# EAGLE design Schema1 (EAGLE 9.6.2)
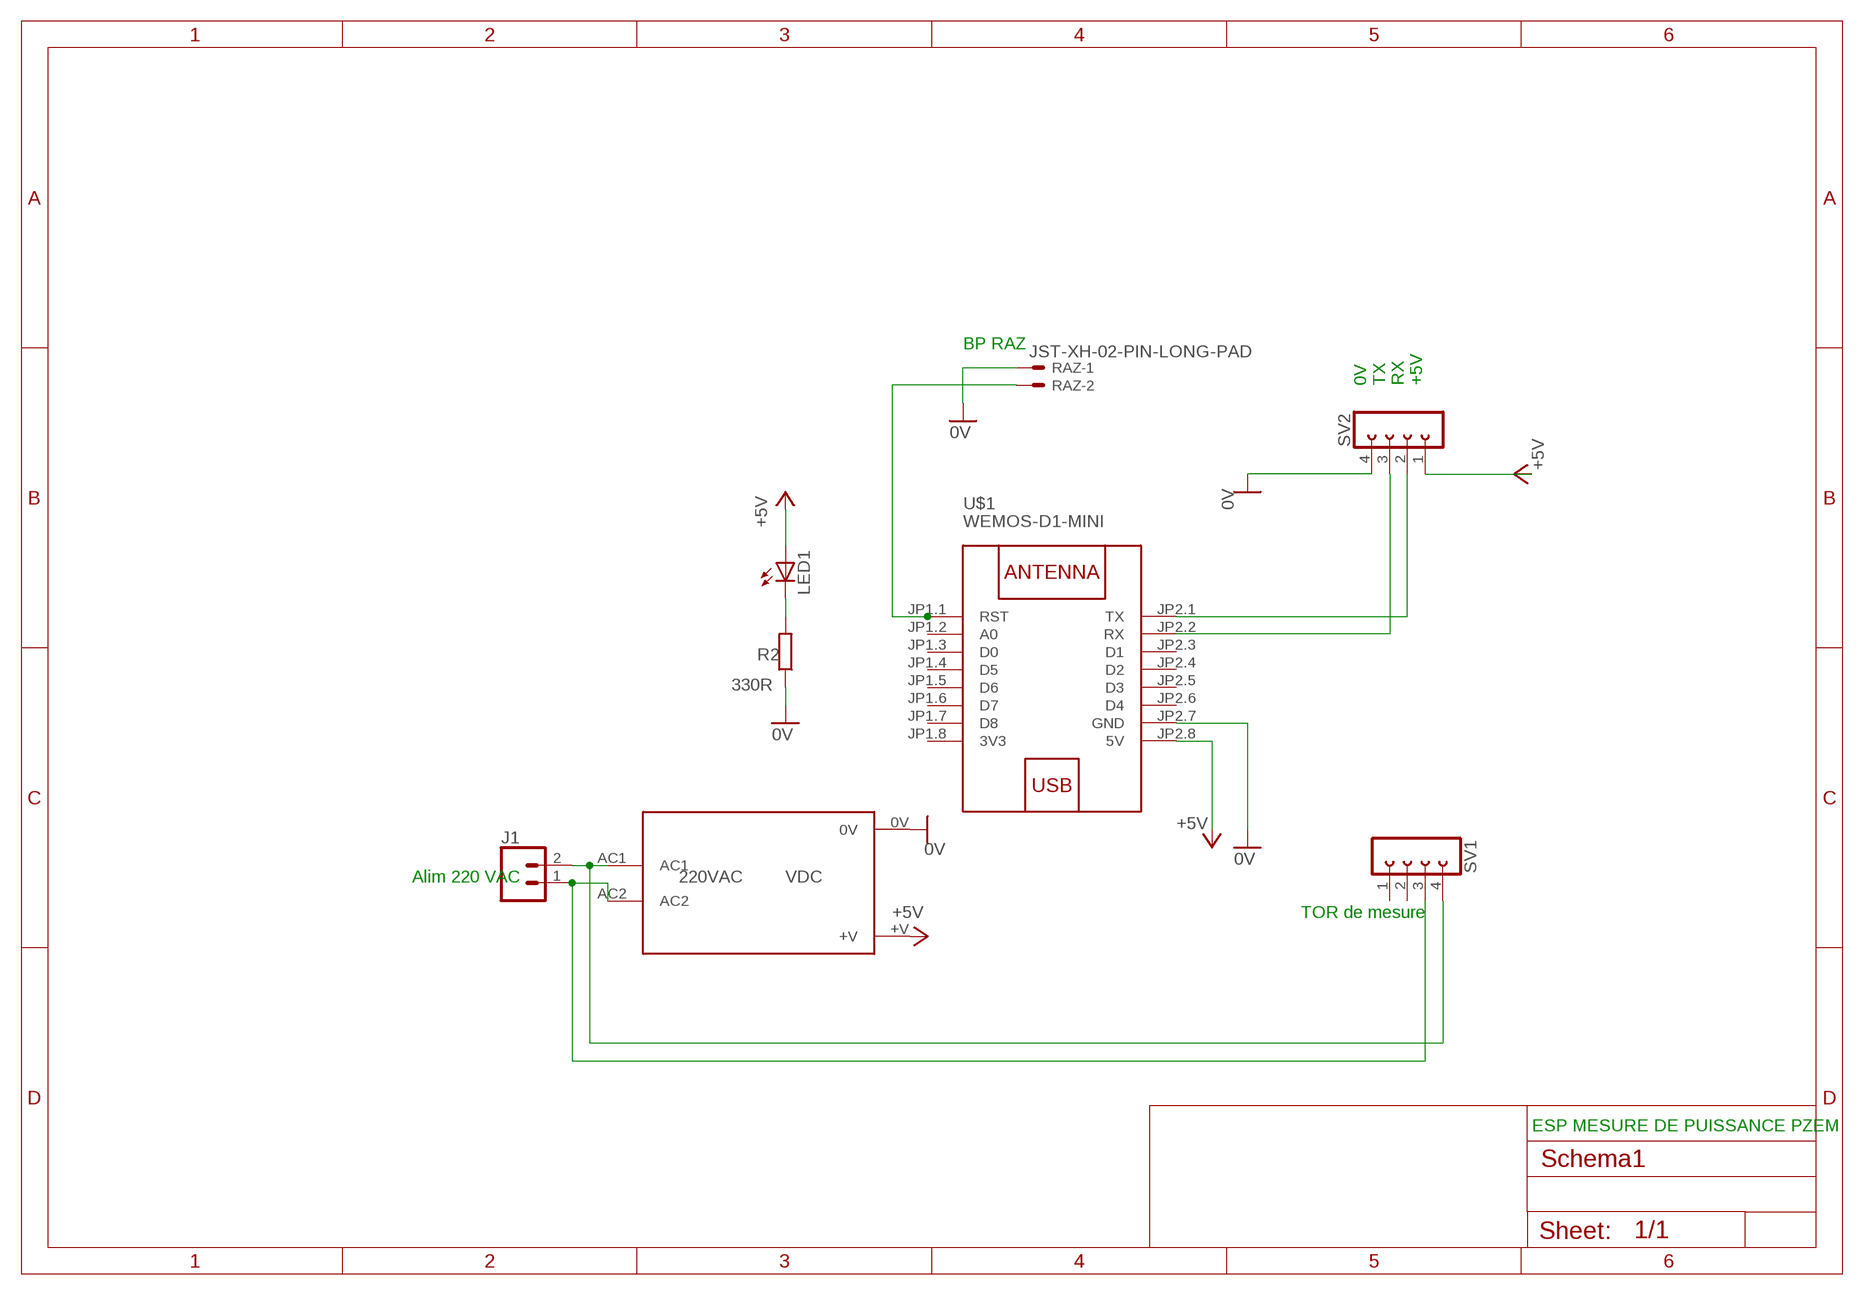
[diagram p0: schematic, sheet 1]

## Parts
J1  CONN_025MM  [BORNIER_A_VIS_2_5.12MM]
LED1  LED5MM_F  [LED5MM]
R2  330R  R-EU_0207/10  [0207/10]
RAZ  JST-XH-02-PIN-LONG-PAD  [JST-XH-02-PACKAGE-LONG-PAD]
SV1  FE04-1  [FE04-1]
SV2  FE04-1  [FE04-1]
U$1  WEMOS-D1-MINI  [WEMOS-D1-MINI]
U$2  TSP05-5V-3W  [TSP05-VDC-3W]

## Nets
0V: R2.1 RAZ.1 SV2.4 U$1.JP2.7(GND) U$2.0V
+5V: LED1.A SV2.1 U$1.JP2.8(5V) U$2.+V
N$1: J1.1 SV1.3 U$2.AC2
N$2: J1.2 SV1.4 U$2.AC1
N$3: LED1.K(C) R2.2
N$4: SV2.3 U$1.JP2.2(RX)
N$6: SV2.2 U$1.JP2.1(TX)
N$7: RAZ.2 U$1.JP1.1(RST)
Unconnected: SV1.1 SV1.2 U$1.JP1.2(A0) U$1.JP1.3(D0) U$1.JP1.4(D5) U$1.JP1.5(D6) U$1.JP1.6(D7) U$1.JP1.7(D8) U$1.JP2.3(D1) U$1.JP2.4(D2) U$1.JP2.5(D3) U$1.JP2.6(D4)

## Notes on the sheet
- BP RAZ
- 0V
  TX
  RX
  +5V
- Alim 220 VAC
- TOR de mesure
- ESP MESURE DE PUISSANCE PZEM

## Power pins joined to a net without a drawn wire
3V3: U$1.JP1.8(3V3)

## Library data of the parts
J1 = 04_Remy:CONN_02: Multi connection point. Often used as Generic Header-pin footprint for 0.1 inch spaced/style header connections; SF_SKU: PRT-08432
LED1 = _Remy:LED: LEDS
R2 = _Remy:R-EU_: RESISTOR, European symbol
RAZ = con-JST XH Connectors v1-0:JST-XH-02-PIN: JST XH Connector 2 Pin
SV1 SV2 = 04_Remy:FE04-1: FEMALE HEADER
U$1 = _Remy:WEMOS-D1-MINI: WEMOS D1 mini: Mini Wi-Fi Board based on ESP-8266 device More details can be found here: https://www.wemos.cc/product/d1-mini.html Click here to find device on ebay.com
U$2 = 04_Remy:TSP05-5V-3W

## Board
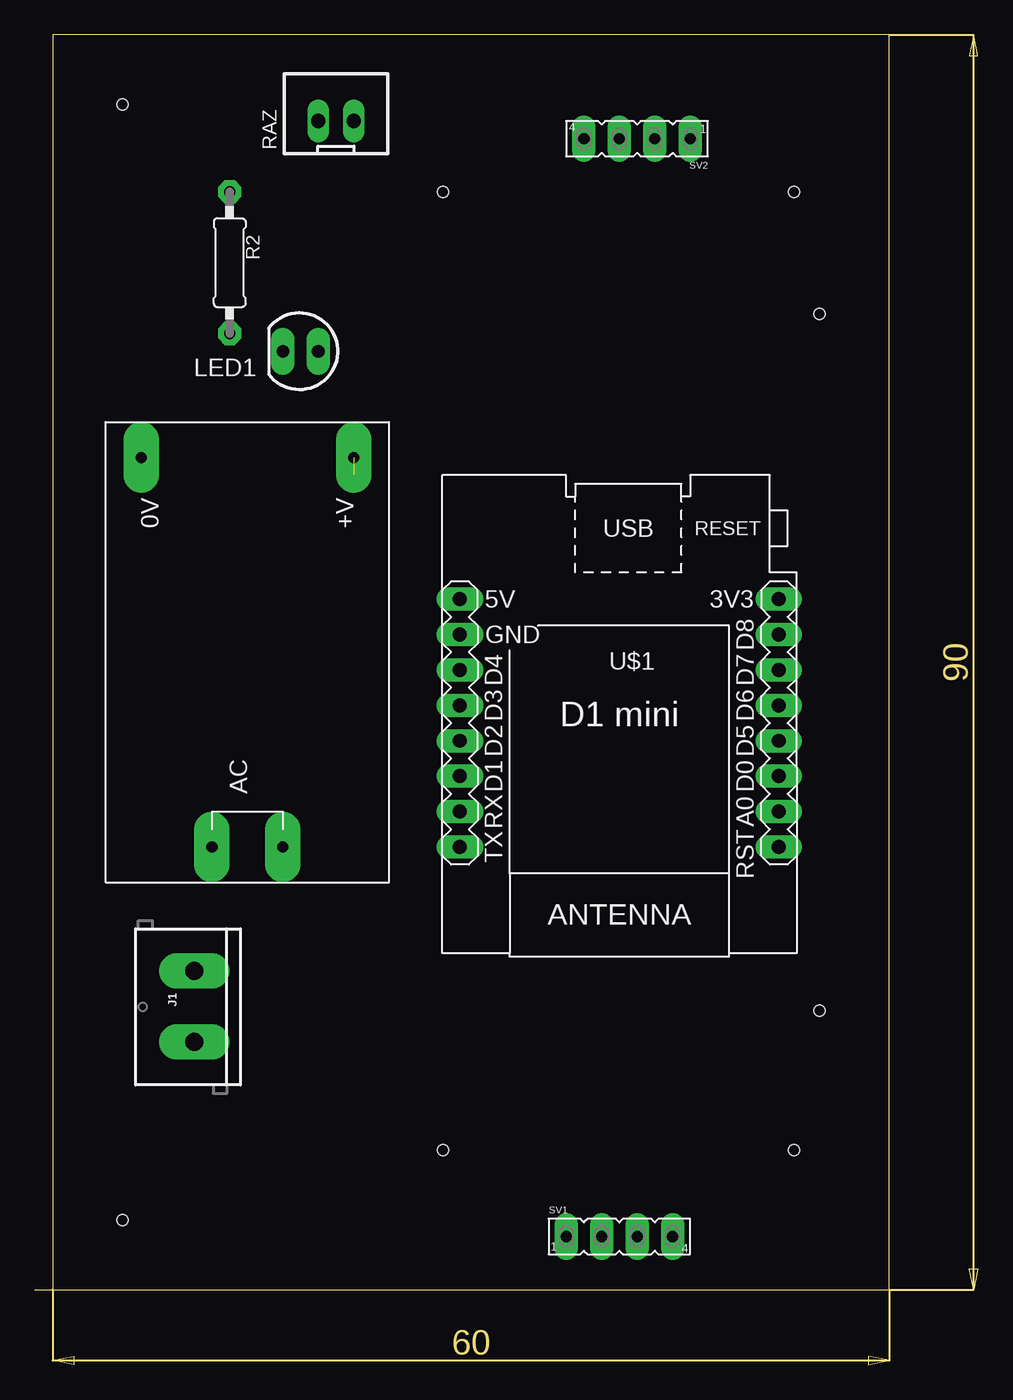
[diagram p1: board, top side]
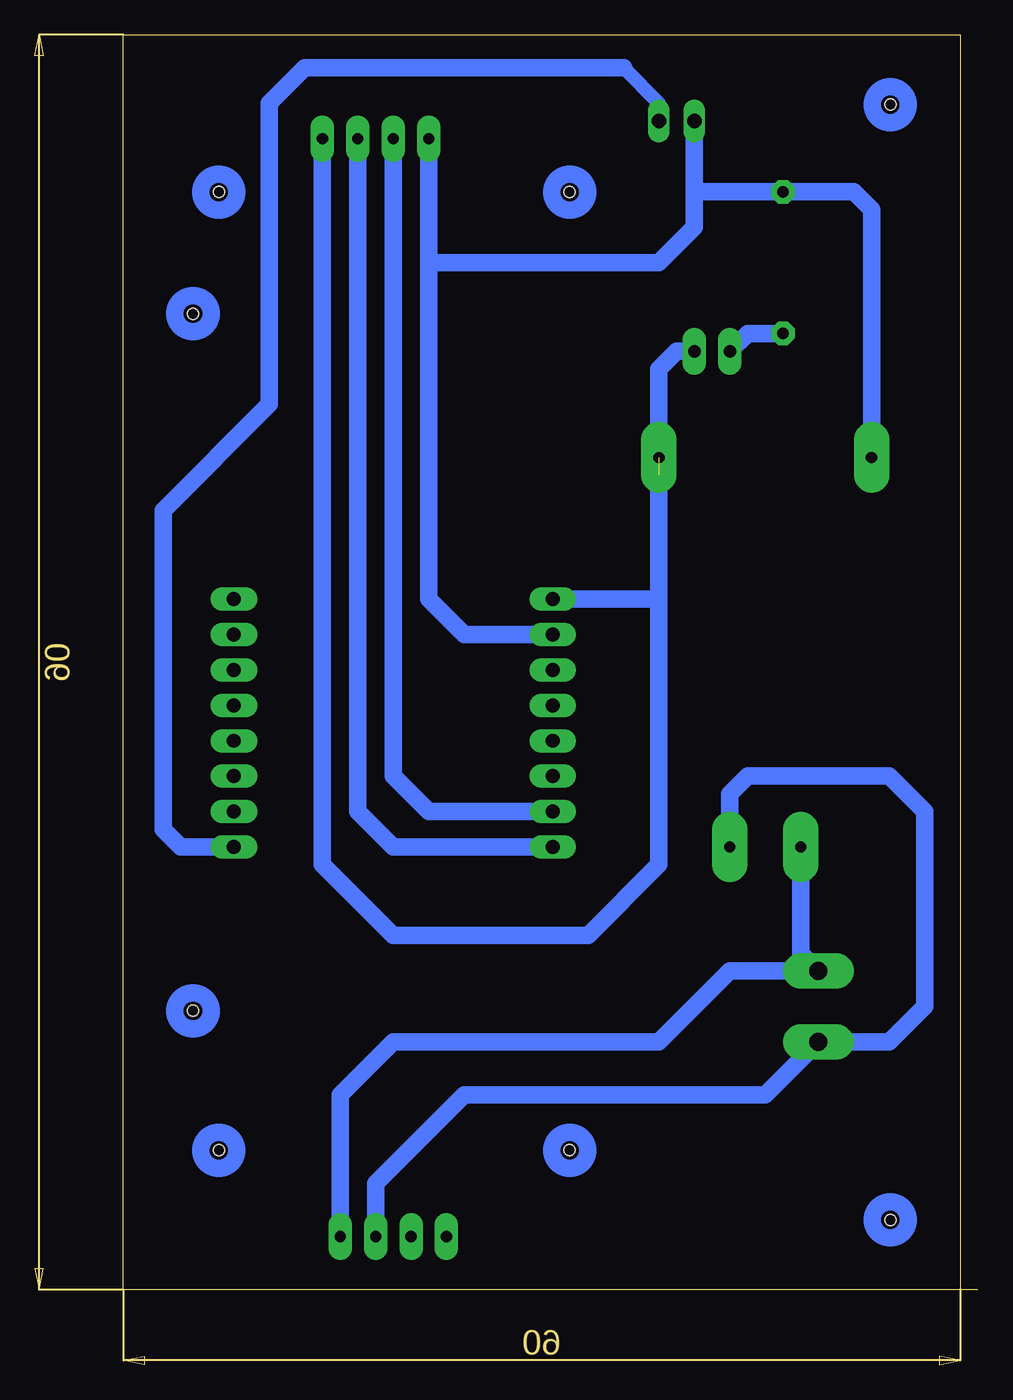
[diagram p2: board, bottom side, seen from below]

Size 67.61 x 95.38 mm. Coordinates in mm from the lower left corner, seen from the top.
Outline: 0,5.38 1.27,5.38
Outline: 1.27,5.38 61.27,5.38 61.27,95.38 1.27,95.38 1.27,5.38
Copper layers (1*16): Top 0.035mm / dielectric 1.5mm / Bottom 0.035mm
Design rules "default": minimum track width 6mil, minimum drill 0.35mm, track to track 6mil, track to pad 6mil, pad to pad 6mil, via to via 6mil, smd to smd 6mil, copper to edge 40mil, drill to drill 6mil, minimum pad ring 10mil, minimum via ring 8mil, stop-mask expansion 4mil, vias tented up to drill 0mil, thermal gap 10mil
Holes 0.8 mm at 6.27,90.38 56.27,75.38 6.27,10.38 56.27,25.38 54.42,15.38 29.27,15.38 29.27,84.1 54.42,84.1

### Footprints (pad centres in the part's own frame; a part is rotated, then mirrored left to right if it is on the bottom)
BORNIER_A_VIS_2_5.12MM = drill 1.3 pad 2.54 long: 1 -2.54,0; 2 2.54,0
LED5MM = drill 0.9 pad 1.676 long: A -1.27,0; K 1.27,0
0207/10 = drill 0.813 pad 1.676 octagon: 1 -5.08,0; 2 5.08,0
JST-XH-02-PACKAGE-LONG-PAD = drill 1.016 long: 1 -1.27,0; 2 1.27,0
FE04-1 = drill 0.8 pad 1.676 long: 1 -3.81,0; 2 -1.27,0; 3 1.27,0; 4 3.81,0
WEMOS-D1-MINI = drill 1 pad 1.676 long: JP1.1 -11.43,10.16; JP1.2 -11.43,7.62; JP1.3 -11.43,5.08; JP1.4 -11.43,2.54; JP1.5 -11.43,0; JP1.6 -11.43,-2.54; JP1.7 -11.43,-5.08; JP1.8 -11.43,-7.62; JP2.1 11.43,10.16; JP2.2 11.43,7.62; JP2.3 11.43,5.08; JP2.4 11.43,2.54; JP2.5 11.43,0; JP2.6 11.43,-2.54; JP2.7 11.43,-5.08; JP2.8 11.43,-7.62
TSP05-VDC-3W = drill 0.8 pad 2.54 long: 0V 13.97,7.62; +V 13.97,-7.62; AC1 -13.97,2.54; AC2 -13.97,-2.54

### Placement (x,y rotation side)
J1  11.43,25.7 90 top
LED1  19.05,72.69 180 top
R2  13.97,79.04 270 top
RAZ  21.59,89.2 0 top
SV1  41.91,9.19 0 top
SV2  43.18,87.93 180 top
U$1  41.91,47.29 180 top
U$2  15.24,51.1 90 top

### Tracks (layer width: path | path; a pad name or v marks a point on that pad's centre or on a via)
0V
  Bottom 1.016: 8.89,84.12 R2.1 20.32,84.12 | RAZ.1 20.32,84.12 | 39.37,77.77 39.37,79.04 SV2.4 | 20.32,84.12 20.32,81.58
  Bottom 1.27: 20.32,84.12 8.89,84.12 7.62,82.85 U$2.0V | RAZ.1 20.32,81.58 22.86,79.04 39.37,79.04 | SV2.4 39.37,77.77 39.37,54.91 36.83,52.37 U$1.JP2.7
+5V  (1 unrouted)
  Bottom 1.016: 29.21,54.91 U$1.JP2.8
  Bottom 1.27: LED1.A 21.59,72.69 22.86,71.42 22.86,63.8 | U$2.+V 22.86,54.91 | 22.86,54.91 22.86,35.86 27.94,30.78 41.91,30.78 46.99,35.86 SV2.1 | U$1.JP2.8 22.86,54.91
N$1
  Bottom 1.27: U$2.AC2 17.78,40.94 16.51,42.21 6.35,42.21 3.81,39.67 3.81,25.7 6.35,23.16 J1.1 | 10.16,23.16 J1.1 | SV1.3 43.18,13 36.83,19.35 15.24,19.35 J1.1
N$2
  Bottom 1.27: U$2.AC1 12.7,29.51 J1.2 17.78,28.24 22.86,23.16 41.91,23.16 45.72,19.35 SV1.4
N$3
  Bottom 1.27: LED1.K 16.51,73.96 R2.2
N$4
  Bottom 1.27: SV2.3 41.91,42.21 39.37,39.67 U$1.JP2.2
N$6
  Bottom 1.27: U$1.JP2.1 41.91,37.13 44.45,39.67 SV2.2
N$7
  Bottom 1.016: 25.4,93.01 22.86,90.47 RAZ.2
  Bottom 1.27: 25.4,93.01 48.26,93.01 50.8,90.47 50.8,68.88 58.42,61.26 58.42,38.4 57.15,37.13 U$1.JP1.1
(copper drawn outside any net)
  shapes: Bottom circle x8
